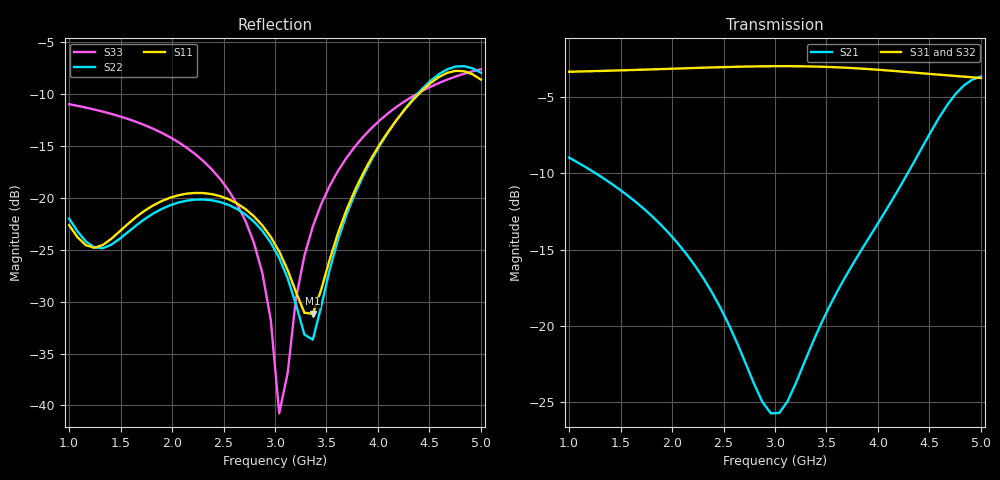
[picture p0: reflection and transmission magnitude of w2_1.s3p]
# GHZ S RI R 50
!Output file by EM3DS 5.12 Built 2
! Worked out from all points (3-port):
!   50 points, 1 GHz to 5 GHz, reference 50 ohm
!   strongest paths, dB at 1 GHz, 1.98 GHz, 3.041 GHz, 4.02 GHz, 5 GHz:
!     S31: -3.3, -3.1, -3.0, -3.2, -3.7
!     S32: -3.4, -3.2, -3.1, -3.3, -4.0
!     S21: -9.0, -14.0, -25.7, -13.1, -3.6
!   lowest |S11| = -31.2 dB at 3.367 GHz (marker M1), VSWR 1.06, Z = 48.3 + j2.13 ohm
!   |S11| at or under -10 dB: start of sweep to 4.396 GHz
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1  0.00193 0.0739  0.05 -0.3529  0.3255 -0.5995
   0.05 -0.3529  0.0124 0.0785  0.3161 -0.5956
   0.3255 -0.5995  0.3161 -0.5956  -0.1991 0.2005
1.326531  -0.0294 0.0515  -0.0576 -0.3003  0.1201 -0.6762
          -0.0576 -0.3003  -0.0172 0.0546  0.1126 -0.6692
          0.1201 -0.6762  0.1126 -0.6692  -0.1593 0.2059
1.734694  -0.0537 0.0681  -0.1346 -0.1994  -0.1631 -0.6739
          -0.1346 -0.1994  -0.04 0.0682  -0.1671 -0.664
          -0.1631 -0.6739  -0.1671 -0.664  -0.0995 0.2006
2.55102  -0.0033 0.0984  -0.0938 -0.0368  -0.6285 -0.3248
         -0.0938 -0.0368  0.00801 0.092  -0.6233 -0.3143
         -0.6285 -0.3248  -0.6233 -0.3143  0.00664 0.1081
2.877551  0.0165 0.0717  -0.0458 -0.0324  -0.7056 -0.0875
          -0.0458 -0.0324  0.0251 0.0646  -0.6969 -0.0791
          -0.7056 -0.0875  -0.6969 -0.0791  0.0162 0.0402
3.040816  0.0153 0.053  -0.0266 -0.0443  -0.7106 0.0395
          -0.0266 -0.0443  0.0226 0.0461  -0.7004 0.0464
          -0.7106 0.0395  -0.7004 0.0464  0.00837 0.00375
3.367347  -0.0168 0.022  -0.00875 -0.0878  -0.6493 0.287
          -0.00875 -0.0878  -0.0118 0.0171  -0.637 0.2902
          -0.6493 0.287  -0.637 0.2902  -0.0359 -0.0633
4.020408  -0.1409 0.1151  -0.0793 -0.2077  -0.2899 0.6283
          -0.0793 -0.2077  -0.1347 0.1185  -0.2771 0.6222
          -0.2899 0.6283  -0.2771 0.6222  -0.2129 -0.1038
4.591837  0.0585 0.3771  -0.4045 -0.2597  0.122 0.6562
          -0.4045 -0.2597  0.0825 0.3853  0.128 0.6395
          0.122 0.6562  0.128 0.6395  -0.3572 0.0125
5  0.3444 0.1383  -0.6327 0.1819  0.3746 0.532
   -0.6327 0.1819  0.3802 0.1255  0.3667 0.5168
   0.3746 0.532  0.3667 0.5168  -0.3875 0.1525
